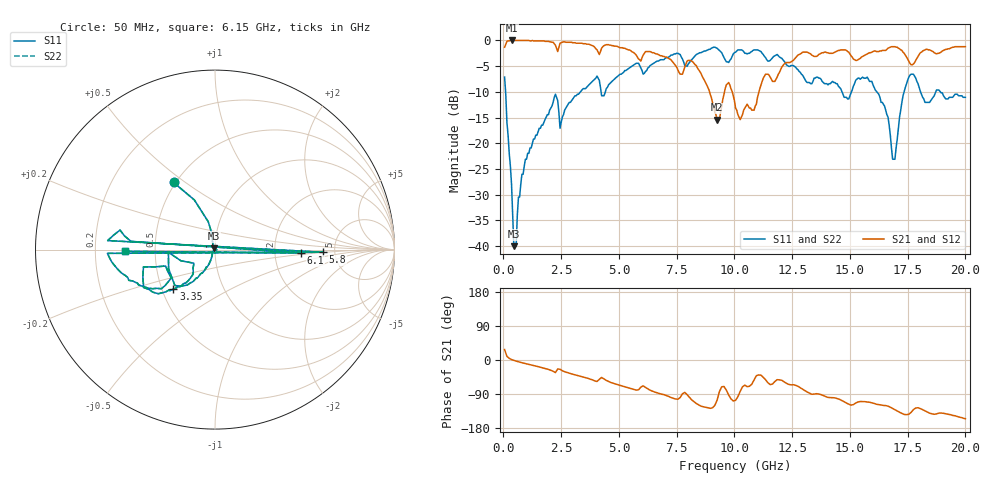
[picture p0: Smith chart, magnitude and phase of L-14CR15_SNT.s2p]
#	mhz	s	ma	r	50
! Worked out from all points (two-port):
!   400 points, 50 MHz to 20 GHz, reference 50 ohm
!   highest |S21| = 0.00 dB at 350 MHz (marker M1); lowest = -15.4 dB at 9.25 GHz (marker M2)
!   |S21| within 3 dB of the highest: start of sweep to 5.77 GHz; 17.96 GHz to end of sweep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
!   lowest |S11| = -40.0 dB at 450 MHz (marker M3), VSWR 1.02, Z = 49.3 + j0.683 ohm
!   |S11| at or under -10 dB: 93.12 MHz to 3.331 GHz (3.238 GHz wide, 189 % of centre); 16.17 GHz to 17.34 GHz (1.175 GHz wide, 7.01 % of centre); 18.92 GHz to end of sweep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
!   |S22| runs from -40.0 to -1.3 dB; largest |S21 - S12| = 0
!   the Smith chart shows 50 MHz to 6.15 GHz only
!   S11 on the Smith chart (normalised r, x): 50 MHz: 0.49, +0.45; 3.35 GHz: 0.57, -0.28; 5.8 GHz: 3.99, -0.18; 6.1 GHz: 2.84, -0.14; 6.15 GHz: 0.33, -0.01
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50  0.44 121.7  0.86 27.6  0.86 27.6  0.44 121.7
350  0.04 108.8  1 1.2  1 1.2  0.04 108.8
450  0.01 136.1  1 -1.0  1 -1.0  0.01 136.1
1300  0.11 -115.2  0.99 -14.6  0.99 -14.6  0.11 -115.2
3350  0.32 -136.4  0.94 -43.2  0.94 -43.2  0.32 -136.4
3400  0.33 -137.1  0.94 -44.0  0.94 -44.0  0.33 -137.1
5750  0.6 -178.0  0.72 -79.5  0.72 -79.5  0.6 -178.0
5800  0.6 -1.4  0.69 -79.1  0.69 -79.1  0.6 -1.4
5850  0.6 175.2  0.66 -78.6  0.66 -78.6  0.6 175.2
6050  0.47 174.4  0.72 -68.3  0.72 -68.3  0.47 174.4
6100  0.48 -2.2  0.75 -70.3  0.75 -70.3  0.48 -2.2
6150  0.5 -178.9  0.78 -72.4  0.78 -72.4  0.5 -178.9
6450  0.59 -180.0  0.76 -82.3  0.76 -82.3  0.59 -180.0
6500  0.6 -0.8  0.76 -83.4  0.76 -83.4  0.6 -0.8
6550  0.61 178.4  0.75 -84.6  0.75 -84.6  0.61 178.4
6700  0.63 175.1  0.73 -87.5  0.73 -87.5  0.63 175.1
9250  0.84 102.4  0.17 -106.0  0.17 -106.0  0.84 102.4
10050  0.77 107.6  0.22 -106.5  0.22 -106.5  0.77 107.6
13350  0.38 49.0  0.72 -90.4  0.72 -90.4  0.38 49.0
16700  0.15 -8.6  0.85 -123.1  0.85 -123.1  0.15 -8.6
17600  0.46 53.3  0.6 -140.6  0.6 -140.6  0.46 53.3
20000  0.28 -67.7  0.87 -154.9  0.87 -154.9  0.28 -67.7
